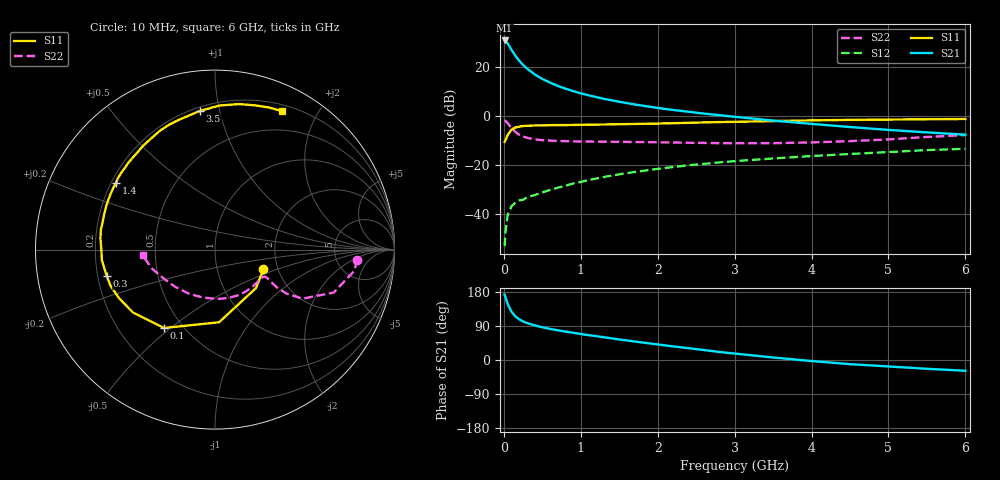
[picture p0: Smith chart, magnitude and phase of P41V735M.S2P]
! SIEMENS Small Signal Semiconductors
! BFP182
! Si NPN RF Bipolar Junction Transistor in SOT143
! VCE = 1.75 V  IC = 35 mA
! Common Emitter S-Parameters:  March  1996
# GHz  S  MA  R  50
!  f  S11  S21  S12  S22
! GHz  MAG  ANG  MAG  ANG  MAG  ANG  MAG  ANG
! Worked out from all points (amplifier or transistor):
!   36 points, 10 MHz to 6 GHz, reference 50 ohm
!   highest |S21| = 30.7 dB at 10 MHz (marker M1)
!   |S21| within 3 dB of that: start of sweep to 84.22 MHz
!   unconditionally stable (mu >= 1): start of sweep to 27.24 MHz; 207.1 MHz to end of sweep
!   at 250 MHz: K = 1.16, MAG = 25.1 dB, |S12| = -34.2 dB
!   at 1.4 GHz: K = 1.92, MAG = 9.8 dB, |S12| = -24.4 dB
!   at 6 GHz: K = 1.37, MAG = -0.7 dB, |S12| = -13.5 dB
!   S11 on the Smith chart (normalised r, x): 10 MHz: 1.68, -0.40; 100 MHz: 0.40, -0.48; 300 MHz: 0.24, -0.11; 1.4 GHz: 0.22, +0.29; 3.5 GHz: 0.22, +0.87; 6 GHz: 0.27, +1.56
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0.01  0.2915 -22.2  34.09 173.0  0.0022 70.4  0.7944 -4.1
0.02  0.3132 -43.2  33.65 166.3  0.0042 72.6  0.7848 -8.7
0.05  0.4055 -86.8  29.74 147.7  0.0095 64.1  0.7035 -19.9
0.1  0.5206 -123.0  21.92 127.3  0.0144 48.7  0.5589 -29.3
0.15  0.5757 -142.4  16.63 115.1  0.0169 43.1  0.466 -31.6
0.2  0.599 -153.0  13.17 107.3  0.0188 45.7  0.4098 -31.5
0.25  0.6159 -160.8  10.83 101.7  0.0194 44.9  0.3763 -30.6
0.3  0.6207 -166.2  9.152 97.8  0.0218 46.8  0.3551 -29.7
0.4  0.633 -174.6  6.977 91.3  0.0242 49.8  0.3303 -28.5
0.5  0.6336 179.6  5.61 86.3  0.0274 51.5  0.3174 -28.4
0.6  0.6416 174.3  4.727 82.1  0.0307 54.0  0.3109 -29.0
0.7  0.6455 169.9  4.042 78.4  0.0341 55.6  0.3066 -30.1
0.8  0.6446 166.1  3.559 75.0  0.0374 56.9  0.3033 -31.4
1.1  0.6555 155.4  2.61 65.6  0.0488 58.1  0.2976 -36.7
1.4  0.6651 146.1  2.063 57.2  0.0601 58.2  0.295 -42.9
1.7  0.6786 137.4  1.694 48.8  0.0715 56.6  0.2904 -50.0
2.2  0.7038 124.6  1.31 35.9  0.09 53.1  0.285 -63.0
2.8  0.7416 110.1  1.025 21.3  0.1117 47.5  0.2762 -80.6
3.5  0.7774 96.2  0.796 6.6  0.1346 40.7  0.2756 -104.1
4.5  0.8218 80.6  0.588 -11.0  0.166 31.0  0.3037 -136.9
5.5  0.8466 69.3  0.457 -23.2  0.1994 21.3  0.3691 -163.8
6  0.8574 64.2  0.411 -28.4  0.2118 15.7  0.4038 -175.5
